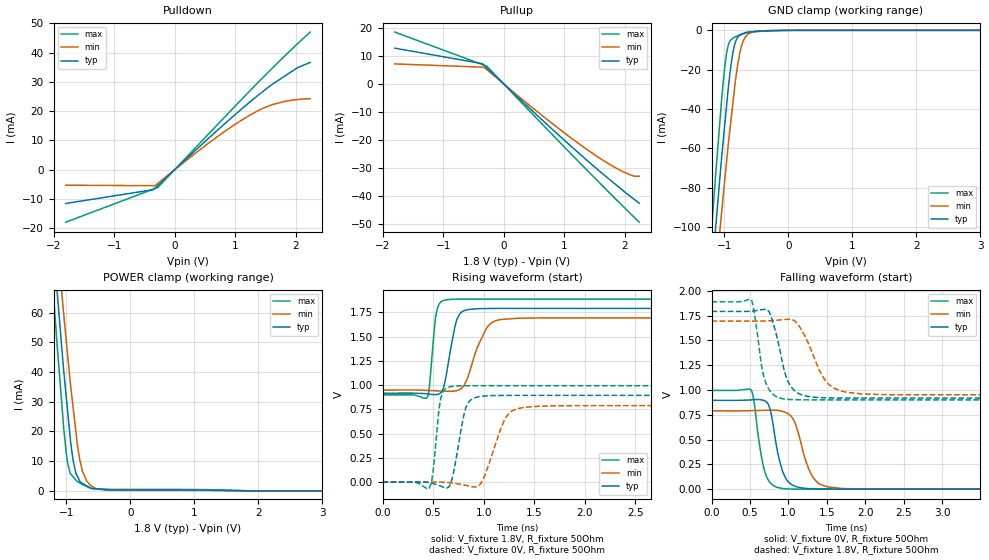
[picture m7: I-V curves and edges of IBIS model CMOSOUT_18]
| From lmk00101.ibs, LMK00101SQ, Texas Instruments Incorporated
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|   Model CMOSOUT_18
[Model]   CMOSOUT_18
Model_type   3-state
Polarity   Non-Inverting
Vmeas = .9
Vref = .9
Cref = 15pF
Rref = 50
|   typ   min   max
|   Nom   Strong   Weak
C_comp   0.4977p   0.4681p   0.5375p
|Output in High
|C_Comp high   0.4977p   0.4681p   0.5375p
|Output in low
|C_Comp low   0.9197p   0.9197p   0.9197p
|Output disabled
|C_Comp disabled   0.8920p   0.8648p   0.9197p
[Voltage Range]   1.8   1.7   1.9
[Temperature Range]   45   125   -40
[Pullup Reference]   1.8   1.7   1.9
[Pulldown Reference]   0   0   0
[Power Clamp Reference]   1.8   1.7   1.9
[GND Clamp Reference]   0   0   0
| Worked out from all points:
|   slope of the pulldown table from 0 to 0.27 V, typ, clamps not added: 51.9 ohm
|   slope of the pullup table from 0 to 0.27 V, typ, clamps not added: 48.9 ohm
|   GND clamp passes 1 mA (typ) near -0.65 V on its own axis
|   POWER clamp passes 1 mA (typ) near -0.63 V on its own axis
|   falling waveform, V_fixture 0V, R_fixture 50Ohm: 20-80 % time 139ps typ, 189ps min, 117ps max; typ from 0.896 V to 0 V
|   rising waveform, V_fixture 1.8V, R_fixture 50Ohm: 20-80 % time 91.4ps typ, 160ps min, 50.4ps max; typ from 0.918 V to 1.79 V
|   rising waveform, V_fixture 0V, R_fixture 50Ohm: 20-80 % time 93ps typ, 160ps min, 55.5ps max; typ from 0 V to 0.896 V
|   falling waveform, V_fixture 1.8V, R_fixture 50Ohm: 20-80 % time 168ps typ, 264ps min, 122ps max; typ from 1.79 V to 0.918 V
[Pulldown]
|   Voltage   I(typ)   I(min)   I(max)
-1.8V     -11.51mA   -5.265mA   -17.89mA
-349.9mV  -6.781mA   -5.432mA   -6.592mA
-323.7mV  -6.272mA   -5.435mA   -6.387mA
-277.1mV  -5.369mA   -4.65mA    -6.024mA
211.8mV   4.074mA    3.498mA    4.602mA
643.8mV   12.26mA    10.33mA    13.97mA
967.8mV   18.23mA    15.05mA    20.99mA
1.292V    23.91mA    19.19mA    27.92mA
1.616V    29.16mA    22.24mA    34.67mA
1.832V    32.1mA     23.37mA    39.04mA
2.026V    34.74mA    23.95mA    42.85mA
2.242V    36.65mA    24.22mA    46.97mA
[GND Clamp]
|   Voltage   I(typ)   I(min)   I(max)
-1.8V     -376.9mA   -373.2mA   -387.4mA
-1.256V   -148.1mA   -168.6mA   -126.6mA
-1.148V   -104.8mA   -129.4mA   -78.18mA
-1.045V   -65.33mA   -93.14mA   -35.99mA
-979mV    -42.98mA   -71.29mA   -14.75mA
-938.5mV  -29.26mA   -57.82mA   -7.52mA
-907.1mV  -20.28mA   -48.68mA   -5.286mA
-837.2mV  -7.006mA   -28.45mA   -3.404mA
-788.1mV  -3.388mA   -16.76mA   -2.744mA
-720.6mV  -1.739mA   -6.632mA   -1.978mA
-531.8mV  -647.2uA   -497.5uA   -705.5uA
3.595V    0A         0A         0A
[Pullup]
|   Voltage   I(typ)   I(min)   I(max)
-1.8V     12.77mA    7.132mA    18.52mA
-349.9mV  7.219mA    5.964mA    6.895mA
-323.7mV  6.676mA    5.943mA    6.685mA
-277.1mV  5.714mA    5.084mA    6.311mA
643.8mV   -13.04mA   -11.45mA   -14.55mA
1.4V      -27.76mA   -23.81mA   -31.34mA
1.616V    -31.78mA   -26.96mA   -36.06mA
1.94V     -37.56mA   -31.06mA   -43.05mA
2.156V    -41.26mA   -33.03mA   -47.66mA
2.242V    -42.69mA   -33.03mA   -49.49mA
[POWER Clamp]
|   Voltage   I(typ)   I(min)   I(max)
-1.8V     254.5mA    252.4mA    261.3mA
-1.256V   97.65mA    112.3mA    82.96mA
-1.148V   68.07mA    85.06mA    50.1mA
-1.045V   41.32mA    60.3mA     22.14mA
-979mV    26.65mA    45.56mA    9.355mA
-934.1mV  16.71mA    35.59mA    5.751mA
-893.6mV  10.24mA    27.99mA    4.731mA
-828.6mV  4.973mA    15.8mA     3.194mA
-757.3mV  2.693mA    7.473mA    2.225mA
-626.1mV  958.6uA    1.931mA    1.035mA
-323.7mV  326.9uA    211.2uA    541.1uA
3.595V    0A         0A         0A
[Ramp]
R_load = 50
|   typ   min   max
dV/dt_r   0.524391/9.13005e-11   0.446809/1.58318e-10   0.593037/5.03823e-11
dV/dt_f   0.537305/1.38706e-10   0.473859/1.88214e-10   0.597179/1.16694e-10
[Falling Waveform]
V_fixture = 0V
V_fixture_min = 0V
V_fixture_max = 0V
R_fixture = 50Ohm
C_fixture = 0F
|   Time   V(typ)   V(min)   V(max)
0s        895.5mV    789.8mV    995.3mV
515ps     899.7mV    791.3mV    1V
689ps     891.7mV    794.5mV    185.3mV
761ps     804.1mV    796.3mV    66.62mV
873ps     325mV      792.3mV    14.04mV
934ps     160mV      781.9mV    5.897mV
1.03ns    52.18mV    739.3mV    1.483mV
1.3ns     3.655mV    145.3mV    35.25uV
1.502ns   495.3uV    24.96mV    2.954uV
4.999ns   6.526nV    32.08nV    6.706nV
[Rising Waveform]
V_fixture = 1.8V
V_fixture_min = 1.7V
V_fixture_max = 1.9V
R_fixture = 50Ohm
C_fixture = 0F
|   Time   V(typ)   V(min)   V(max)
0s        918mV      950mV      900mV
442ps     910.9mV    946.4mV    874.9mV
463ps     908.4mV    945.5mV    985.8mV
532ps     903.6mV    942.6mV    1.746V
626ps     1.083V     938.2mV    1.88V
733ps     1.671V     944.1mV    1.887V
849ps     1.78V      1.102V     1.888V
1.025ns   1.791V     1.582V     1.888V
1.178ns   1.792V     1.679V     1.888V
4.999ns   1.792V     1.695V     1.888V
[Rising Waveform]
V_fixture = 0V
V_fixture_min = 0V
V_fixture_max = 0V
R_fixture = 50Ohm
C_fixture = 0F
|   Time   V(typ)   V(min)   V(max)
0s        6.526nV    31.19nV    6.706nV
460ps     -4.768mV   1.571mV    -63.49mV
497ps     -13.24mV   1.555mV    92.74mV
574ps     -39.41mV   784.4uV    856.5mV
675ps     -8.931mV   -6.916mV   986.1mV
822ps     763mV      -31.72mV   994.8mV
942ps     879.4mV    -43.49mV   995.2mV
1.217ns   894.9mV    664.5mV    995.3mV
1.393ns   895.4mV    771mV      995.3mV
4.999ns   895.5mV    789.8mV    995.3mV
[Falling Waveform]
|Gnd
V_fixture = 1.8V
V_fixture_min = 1.7V
V_fixture_max = 1.9V
R_fixture = 50Ohm
C_fixture = 0F
|   Time   V(typ)   V(min)   V(max)
0s        1.792V     1.695V     1.888V
515ps     1.793V     1.694V     1.911V
687ps     1.813V     1.695V     1.116V
774ps     1.741V     1.698V     976.4mV
901ps     1.356V     1.706V     915.9mV
989ps     1.095V     1.712V     905.4mV
1.12ns    970.3mV    1.665V     901.2mV
1.476ns   921mV      1.099V     900.1mV
1.749ns   918.5mV    977.4mV    900mV
4.999ns   918mV      950mV      900mV
